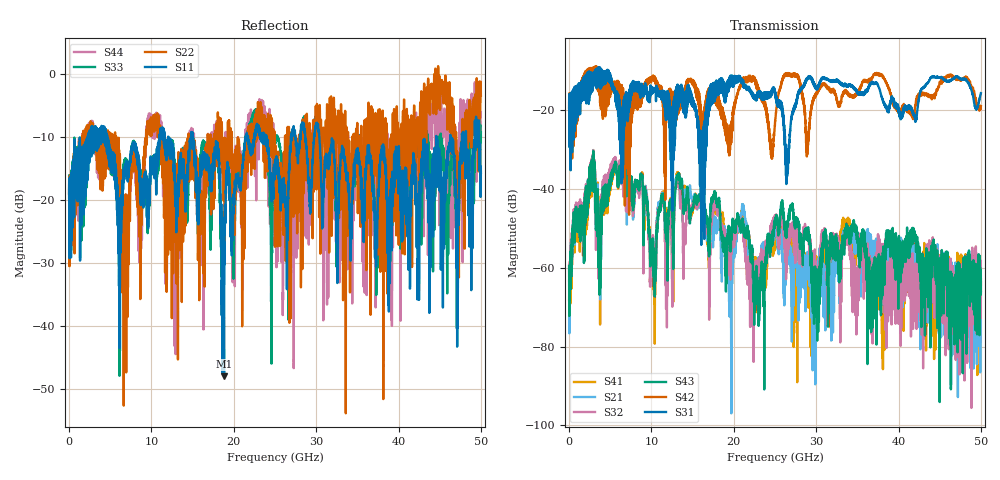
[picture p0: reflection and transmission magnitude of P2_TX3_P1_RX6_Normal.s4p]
!Keysight Technologies,N5225B,MY57041031,A.13.20.10
!Date: Friday, May 31, 2019 11:23:19
!Correction: S11(Full 4 Port(1,2,3,4))
!S12(Full 4 Port(1,2,3,4))
!S13(Full 4 Port(1,2,3,4))
!S14(Full 4 Port(1,2,3,4))
!S21(Full 4 Port(1,2,3,4))
!S22(Full 4 Port(1,2,3,4))
!S23(Full 4 Port(1,2,3,4))
!S24(Full 4 Port(1,2,3,4))
!S31(Full 4 Port(1,2,3,4))
!S32(Full 4 Port(1,2,3,4))
!S33(Full 4 Port(1,2,3,4))
!S34(Full 4 Port(1,2,3,4))
!S41(Full 4 Port(1,2,3,4))
!S42(Full 4 Port(1,2,3,4))
!S43(Full 4 Port(1,2,3,4))
!S44(Full 4 Port(1,2,3,4))
!S4P File: Measurements: <S11,S12,S13,S14>,
!<S21,S22,S23,S24>,
!<S31,S32,S33,S34>,
!<S41,S42,S43,S44>:
# Hz S  dB  R 50.0
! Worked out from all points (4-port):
!   5000 points, 10 MHz to 50 GHz, reference 50 ohm
!   strongest paths, dB at 10 MHz, 12.51 GHz, 25.01 GHz, 37.51 GHz, 50 GHz:
!     S31: -19.5, -43.5, -16.1, -13.6, -15.6
!     S42: -19.4, -15.6, -22.8, -10.7, -18.9
!     S43: -59.5, -46.4, -48.0, -63.8, -66.2
!     S32: -59.5, -65.0, -47.2, -51.4, -62.9
!     S21: -63.3, -62.8, -50.7, -55.0, -65.5
!     S41: -68.2, -47.2, -52.4, -58.7, -63.7
!   lowest |S11| = -47.9 dB at 18.82 GHz (marker M1), VSWR 1.01, Z = 49.6 + j0.0694 ohm
!   |S11| at or under -10 dB: 4.63 GHz to 10.95 GHz (6.318 GHz wide, 81.1 % of centre); 15.04 GHz to 21.46 GHz (6.426 GHz wide, 35.2 % of centre); 30.38 GHz to 44.61 GHz (14.22 GHz wide, 37.9 % of centre)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
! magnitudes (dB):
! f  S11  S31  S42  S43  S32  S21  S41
! 10 MHz  -19.6  -19.5  -19.4  -59.5  -59.5  -63.3  -68.2
! 2.85 GHz  -11.6  -12.4  -10.2  -34.9  -34.7  -34.8  -34.8
! 6.89 GHz  -15.8  -16.6  -21.5  -35.3  -40.4  -38.6  -34.1
! 10.31 GHz  -13.3  -14.6  -12.4  -64.8  -58.4  -62.5  -66.7
! 13.17 GHz  -22.6  -15.6  -18.3  -36.6  -38.4  -37.2  -35.9
! 18.82 GHz  -47.9  -13.2  -23.2  -53.4  -50.6  -51.2  -50.9
! 50 GHz  -15.7  -15.6  -18.9  -66.2  -62.9  -65.5  -63.7
